(* Logix 5000 AddOnInstructionDefinition export YAI_Assy_170_120_EIP_Hz; software revision 21.03 *)

ADD_ON_INSTRUCTION YAI_Assy_170_120_EIP_Hz   (* revision 1.0, vendor Yaskawa America, Inc. *)
// YAI Assembly 170 and 120
// Help:
// This add-on instruction is for use with input assemblie 166 and output assemblies 116.
// Node_Input_Assy is defined as the node's input assembly integer array.
// Node_Output_Assy is defined as the node's output assembly integer array.
// Torque limit/reference, torque compensation and torque output variables are only available with A1000.
VAR_IN_OUT
   Node_Input_Assy : AB:ETHERNET_MODULE_INT_24Bytes:I:0; {required}   // Input assembly words
   Node_Output_Assy : AB:ETHERNET_MODULE_INT_24Bytes:O:0; {required}   // Output assembly words
END_VAR
VAR_INPUT
   RunFwd : BOOL; {visible}   // Forward run command
   RunRev : BOOL; {visible}   // Reverse run command
   MFI_3 : BOOL; {visible}   // Multi-function input 3
   MFI_4 : BOOL; {visible}   // Multi-function input 4
   MFI_5 : BOOL; {visible}   // Multi-function input 5
   MFI_6 : BOOL; {visible}   // Multi-function input 6
   MFI_7 : BOOL; {visible}   // Multi-function input 7
   MFI_8 : BOOL; {visible}   // Multi-function input 8
   External_Fault : BOOL;   // External fault command (EF0)
   FaultReset : BOOL; {visible}   // Fault reset command
   MFO_1 : BOOL; {visible}   // Multi-function output (M1-M2 for A/P1000, MA/MB/MC for V1000)
   MFO_2 : BOOL; {visible}   // Multi-function output (M3-M4 for A/P1000, P1 for V1000)
   MFO_3 : BOOL; {visible}   // Multi-function output (M5-M6 for A/P1000, P2 for V1000)
   Freq_Ref : REAL; {visible}   // Frequency reference command in Hz (xx.xx resolution)
   Net_Ref : BOOL;   // Network reference control bit
   Net_Control : BOOL;   // Network start/stop control bit
   Custom_Out_1 : INT; {visible}   // Custom output 1 - F7-23
   Custom_Out_2 : INT; {visible}   // Custom output 2 - F7-24
   Custom_Out_3 : INT; {visible}   // Custom output 3 - F7-25
   Custom_Out_4 : INT;   // Custom output 4 - F7-26
   Custom_Out_5 : INT;   // Custom output 5 - F7-27
   Custom_Out_6 : INT;   // Custom output 6 - F7-28
   Custom_Out_7 : INT;   // Custom output 7 - F7-29
   Custom_Out_8 : INT;   // Custom output 8 - F7-30
   Custom_Out_9 : INT;   // Custom output 9 - F7-31
   Custom_Out_10 : INT;   // Custom output 10 - F7-32
END_VAR
VAR_OUTPUT
   Running : BOOL; {access Read Only, visible}   // Drive running forward status bit
   ZSP : BOOL; {access Read Only, visible}   // Drive zero speed status bit
   RunningRev : BOOL; {access Read Only, visible}   // Drive running reverse status bit
   Reset : BOOL; {access Read Only, visible}   // Drive reset command status bit
   At_Speed : BOOL; {access Read Only, visible}   // Drive at commanded speed status bit
   Ready : BOOL; {access Read Only, visible}   // Drive ready status bit
   Alarm : BOOL; {access Read Only, visible}   // Drive alarm status bit
   Faulted : BOOL; {access Read Only, visible}   // Drive faulted status bit
   OPE : BOOL; {access Read Only}   // OPE alarm/fault present
   UV : BOOL; {access Read Only}   // Drive in UV (undervoltage) state status bit
   NetCtrlStatus : BOOL; {access Read Only, visible}   // Drive network run source status bit (1 = source coming from network)
   MFO_1_Status : BOOL; {access Read Only, visible}   // Drive multi-function output 1 (M1-M2 for A/P1000, MA/MB/MC for V1000) status
   MFO_2_Status : BOOL; {access Read Only, visible}   // Drive multi-function output 1 (M3-M4 for A/P1000, P1 for V1000) status
   MFO_3_Status : BOOL; {access Read Only, visible}   // Drive multi-function output 1 (M5-M6 for A/P1000, P2 for V1000) status
   ZSV : BOOL; {access Read Only, visible}   // Drive zero servo completed status bit
   Motor_Speed : REAL; {access Read Only, visible}   // Motor speed in Hz (xx.xx resolution)
   Freq_Cmd : REAL; {access Read Only, visible}   // Commanded frequency in Hz (xx.xx resolution)
   Output_Freq : REAL; {access Read Only, visible}   // Drive output frequency in Hz (xx.xx resolution)
   Custom_In_1 : INT; {access Read Only, visible}   // Custom input 1 - F7-33
   Custom_In_2 : INT; {access Read Only, visible}   // Custom input 2 - F7-34
   Custom_In_3 : INT; {access Read Only, visible}   // Custom input 3 - F7-35
   Custom_In_4 : INT; {access Read Only}   // Custom input 4 - F7-36
   Custom_In_5 : INT; {access Read Only}   // Custom input 5 - F7-37
   Custom_In_6 : INT; {access Read Only}   // Custom input 6 - F7-38
   Custom_In_7 : INT; {access Read Only}   // Custom input 7 - F7-39
   Custom_In_8 : INT; {access Read Only}   // Custom input 8 -F7-40
   Custom_In_9 : INT; {access Read Only}   // Custom input 9 - F7-41
   Custom_In_10 : INT; {access Read Only}   // Custom input 10 - F7-42
END_VAR
VAR
   FRef_Convert : DINT;
   FOut_Convert : REAL;
   FOut_Temp : REAL;
   TRef_Convert : INT;
   TComp_Convert : INT;
   TOut_Convert : REAL;
   TOut_Temp : REAL;
   IOut_Temp : REAL;
   IOut_Convert : REAL;
   AO1_Convert : INT;
   AO2_Convert : INT;
   Motor_Speed_Temp : REAL;
   Motor_Speed_Convert : REAL;
   Freq_Cmd_Temp : REAL;
   Freq_Cmd_Convert : REAL;
   AI1_Temp : REAL;
   AI1_Convert : REAL;
END_VAR

ROUTINE Logic   (* ladder *)
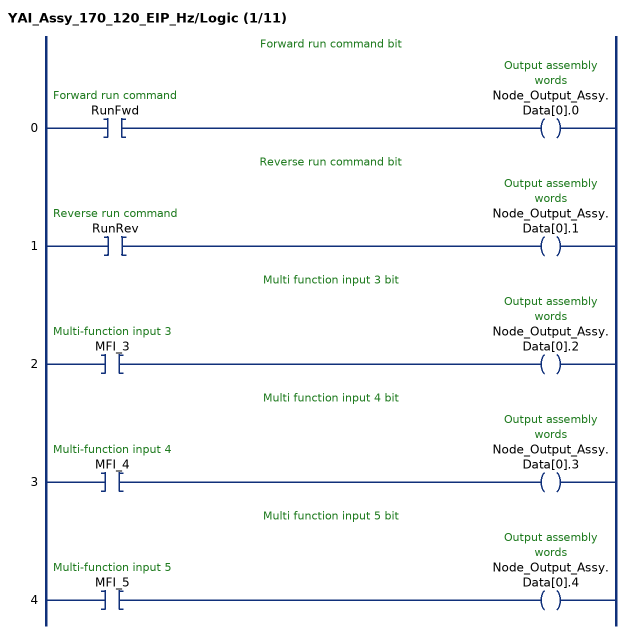
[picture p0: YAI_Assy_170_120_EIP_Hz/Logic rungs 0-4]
   // Forward run command bit
   0: XIC(RunFwd)OTE(Node_Output_Assy.Data[0].0);
   // Reverse run command bit
   1: XIC(RunRev)OTE(Node_Output_Assy.Data[0].1);
   // Multi function input 3 bit
   2: XIC(MFI_3)OTE(Node_Output_Assy.Data[0].2);
   // Multi function input 4 bit
   3: XIC(MFI_4)OTE(Node_Output_Assy.Data[0].3);
   // Multi function input 5 bit
   4: XIC(MFI_5)OTE(Node_Output_Assy.Data[0].4);
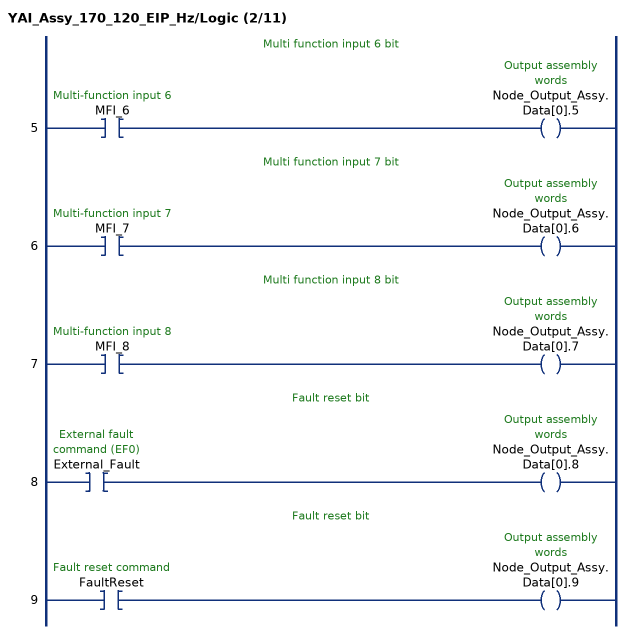
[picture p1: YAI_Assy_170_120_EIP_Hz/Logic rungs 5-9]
   // Multi function input 6 bit
   5: XIC(MFI_6)OTE(Node_Output_Assy.Data[0].5);
   // Multi function input 7 bit
   6: XIC(MFI_7)OTE(Node_Output_Assy.Data[0].6);
   // Multi function input 8 bit
   7: XIC(MFI_8)OTE(Node_Output_Assy.Data[0].7);
   // Fault reset bit
   8: XIC(External_Fault)OTE(Node_Output_Assy.Data[0].8);
   // Fault reset bit
   9: XIC(FaultReset)OTE(Node_Output_Assy.Data[0].9);
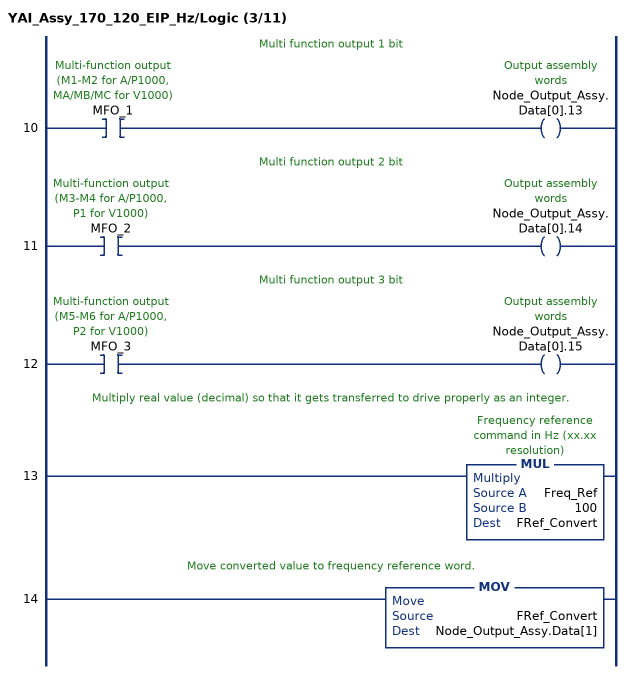
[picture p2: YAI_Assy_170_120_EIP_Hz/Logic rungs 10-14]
   // Multi function output 1 bit
   10: XIC(MFO_1)OTE(Node_Output_Assy.Data[0].13);
   // Multi function output 2 bit
   11: XIC(MFO_2)OTE(Node_Output_Assy.Data[0].14);
   // Multi function output 3 bit
   12: XIC(MFO_3)OTE(Node_Output_Assy.Data[0].15);
   // Multiply real value (decimal) so that it gets transferred to drive properly as an integer.
   13: MUL(Freq_Ref,100,FRef_Convert);
   // Move converted value to frequency reference word.
   14: MOV(FRef_Convert,Node_Output_Assy.Data[1]);
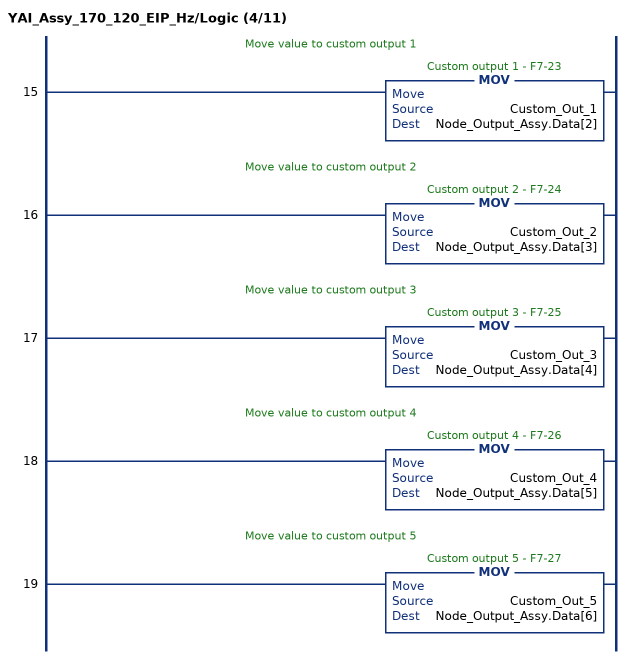
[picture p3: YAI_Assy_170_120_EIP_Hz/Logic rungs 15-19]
   // Move value to custom output 1
   15: MOV(Custom_Out_1,Node_Output_Assy.Data[2]);
   // Move value to custom output 2
   16: MOV(Custom_Out_2,Node_Output_Assy.Data[3]);
   // Move value to custom output 3
   17: MOV(Custom_Out_3,Node_Output_Assy.Data[4]);
   // Move value to custom output 4
   18: MOV(Custom_Out_4,Node_Output_Assy.Data[5]);
   // Move value to custom output 5
   19: MOV(Custom_Out_5,Node_Output_Assy.Data[6]);
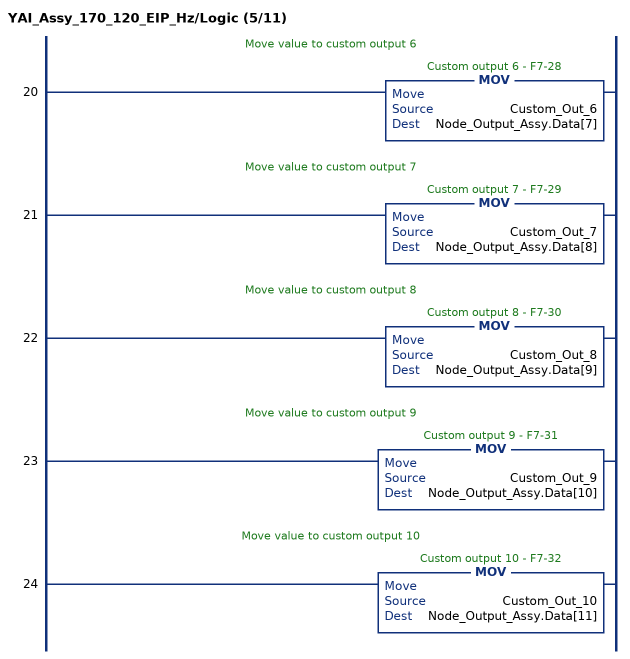
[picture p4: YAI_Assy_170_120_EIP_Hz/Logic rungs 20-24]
   // Move value to custom output 6
   20: MOV(Custom_Out_6,Node_Output_Assy.Data[7]);
   // Move value to custom output 7
   21: MOV(Custom_Out_7,Node_Output_Assy.Data[8]);
   // Move value to custom output 8
   22: MOV(Custom_Out_8,Node_Output_Assy.Data[9]);
   // Move value to custom output 9
   23: MOV(Custom_Out_9,Node_Output_Assy.Data[10]);
   // Move value to custom output 10
   24: MOV(Custom_Out_10,Node_Output_Assy.Data[11]);
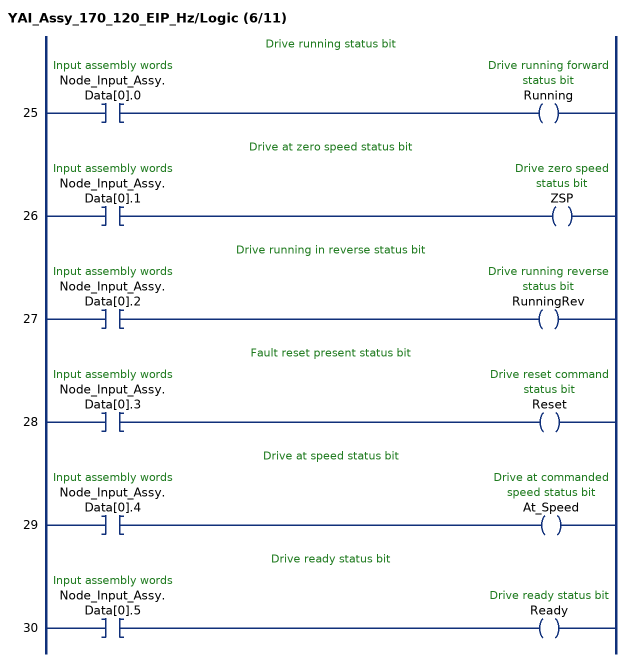
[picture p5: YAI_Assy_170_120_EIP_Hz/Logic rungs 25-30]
   // Drive running status bit
   25: XIC(Node_Input_Assy.Data[0].0)OTE(Running);
   // Drive at zero speed status bit
   26: XIC(Node_Input_Assy.Data[0].1)OTE(ZSP);
   // Drive running in reverse status bit
   27: XIC(Node_Input_Assy.Data[0].2)OTE(RunningRev);
   // Fault reset present status bit
   28: XIC(Node_Input_Assy.Data[0].3)OTE(Reset);
   // Drive at speed status bit
   29: XIC(Node_Input_Assy.Data[0].4)OTE(At_Speed);
   // Drive ready status bit
   30: XIC(Node_Input_Assy.Data[0].5)OTE(Ready);
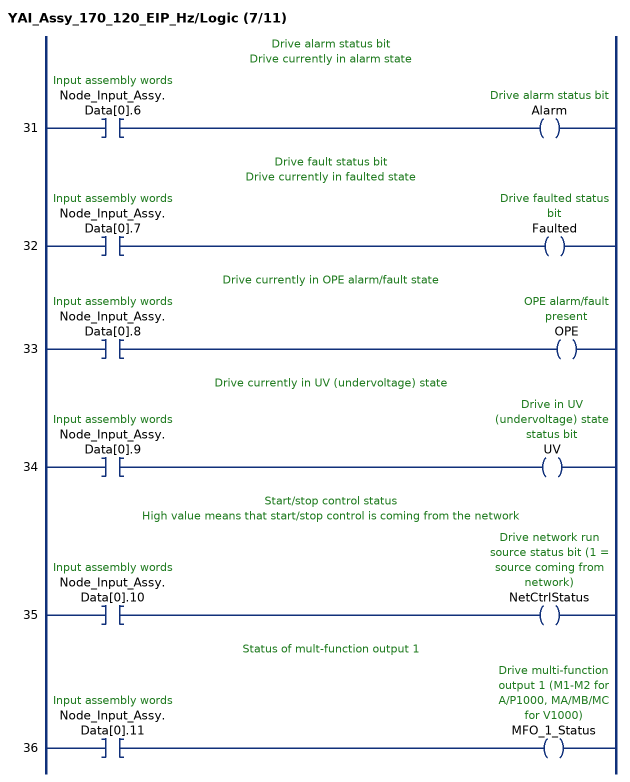
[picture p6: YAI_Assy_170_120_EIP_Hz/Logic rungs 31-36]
   // Drive alarm status bit
   // Drive currently in alarm state
   31: XIC(Node_Input_Assy.Data[0].6)OTE(Alarm);
   // Drive fault status bit
   // Drive currently in faulted state
   32: XIC(Node_Input_Assy.Data[0].7)OTE(Faulted);
   // Drive currently in OPE alarm/fault state
   33: XIC(Node_Input_Assy.Data[0].8)OTE(OPE);
   // Drive currently in UV (undervoltage) state
   34: XIC(Node_Input_Assy.Data[0].9)OTE(UV);
   // Start/stop control status
   // High value means that start/stop control is coming from the network
   35: XIC(Node_Input_Assy.Data[0].10)OTE(NetCtrlStatus);
   // Status of mult-function output 1
   36: XIC(Node_Input_Assy.Data[0].11)OTE(MFO_1_Status);
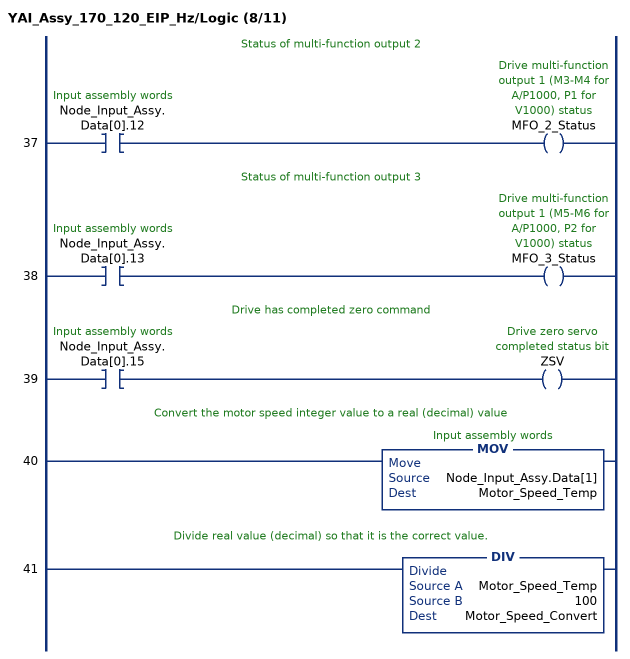
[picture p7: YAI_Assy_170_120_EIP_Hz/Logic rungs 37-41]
   // Status of multi-function output 2
   37: XIC(Node_Input_Assy.Data[0].12)OTE(MFO_2_Status);
   // Status of multi-function output 3
   38: XIC(Node_Input_Assy.Data[0].13)OTE(MFO_3_Status);
   // Drive has completed zero command
   39: XIC(Node_Input_Assy.Data[0].15)OTE(ZSV);
   // Convert the motor speed integer value to a real (decimal) value
   40: MOV(Node_Input_Assy.Data[1],Motor_Speed_Temp);
   // Divide real value (decimal) so that it is the correct value.
   41: DIV(Motor_Speed_Temp,100,Motor_Speed_Convert);
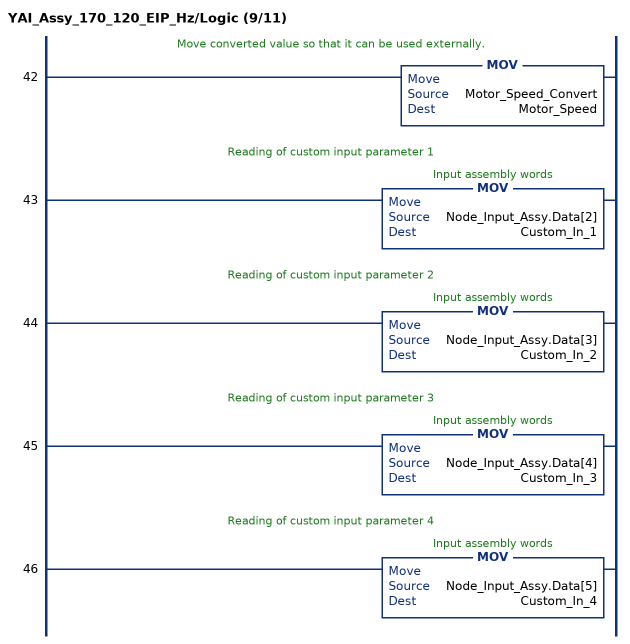
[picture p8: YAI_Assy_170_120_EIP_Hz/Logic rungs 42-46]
   // Move converted value so that it can be used externally.
   42: MOV(Motor_Speed_Convert,Motor_Speed);
   // Reading of custom input parameter 1
   43: MOV(Node_Input_Assy.Data[2],Custom_In_1);
   // Reading of custom input parameter 2
   44: MOV(Node_Input_Assy.Data[3],Custom_In_2);
   // Reading of custom input parameter 3
   45: MOV(Node_Input_Assy.Data[4],Custom_In_3);
   // Reading of custom input parameter 4
   46: MOV(Node_Input_Assy.Data[5],Custom_In_4);
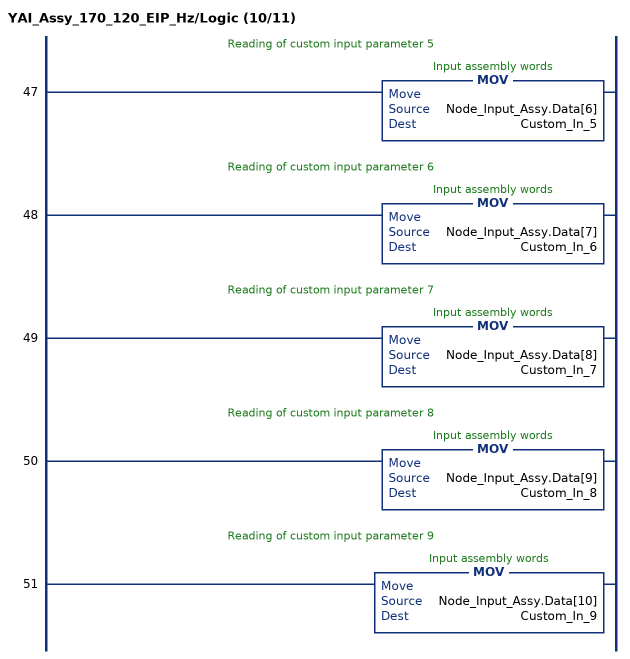
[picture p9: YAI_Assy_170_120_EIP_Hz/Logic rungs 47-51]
   // Reading of custom input parameter 5
   47: MOV(Node_Input_Assy.Data[6],Custom_In_5);
   // Reading of custom input parameter 6
   48: MOV(Node_Input_Assy.Data[7],Custom_In_6);
   // Reading of custom input parameter 7
   49: MOV(Node_Input_Assy.Data[8],Custom_In_7);
   // Reading of custom input parameter 8
   50: MOV(Node_Input_Assy.Data[9],Custom_In_8);
   // Reading of custom input parameter 9
   51: MOV(Node_Input_Assy.Data[10],Custom_In_9);
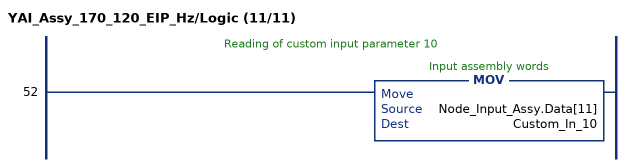
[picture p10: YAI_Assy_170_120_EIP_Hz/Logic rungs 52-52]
   // Reading of custom input parameter 10
   52: MOV(Node_Input_Assy.Data[11],Custom_In_10);
END_ROUTINE
END_ADD_ON_INSTRUCTION
